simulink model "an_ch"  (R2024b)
settings: Solver=ode45  StartTime=0.0  StopTime=2  MaxStep=.01  RelTol=1e-3  AbsTol=1e-3  EnableMultiTasking=on
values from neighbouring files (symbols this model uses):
  den = 1    [ass_appr.m]    (also in simplify.m = a(find(a):max(size(a))); ass_sis.m; ass1_sis.m; myfbode.m = b)
  den_c = 1    [ass_c.m]    (also in ass_sis.m; ass2_cn.m; ass1_sis.m)
  num = b(find(b):max(size(b)))    [simplify.m]    (also in ass_sis.m = 0; ass1_sis.m = 0; myfbode.m = a; mynyq.m = a)
  num_c = 0    [ass_c.m]    (also in ass_sis.m; ass2_cn.m; ass1_sis.m)
  T = 0; end    [ass_appr.m]    (also in ass_sis.m = 0; ass1_sis.m = 0; myfbode.m = rit)
undefined symbols (not defined in the file or in its folder): sfunyst

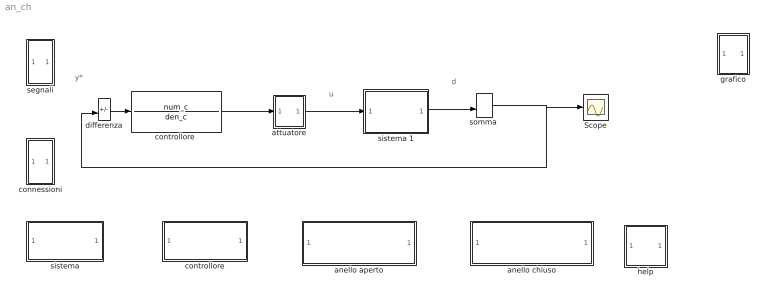
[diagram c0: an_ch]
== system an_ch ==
  note: u
  note: d
  note: y*
  Scope : Scope
  anello aperto : Subsystem
  anello chiuso : Subsystem
  attuatore : Subsystem  mask{upperlimit=inf, lowerlimit=-inf}
      mask prompts: upperlimit "limite superiore"; lowerlimit "limite inferiore"
  connessioni : Subsystem
  controllore : Subsystem
  "controllore " : TransferFcn  Numerator=num_c  Denominator=den_c
  differenza : Sum  Inputs=+-  InputSameDT=on  SaturateOnIntegerOverflow=on
  grafico : Subsystem  Commented=on  mask(Storage scope.){MaskParam1=2, MaskParam2=-10, MaskParam3=10, npts=2000, color='b-/r-/c-./w:/m*/ro/b+'}
      mask prompts: MaskParam1 "Initial Time Range:"; MaskParam2 "Initial y-min:"; MaskParam3 "Initial y-max:"; npts "Storage pts.:"; color "Line type (rgbw-.:xo):"
      mask help: Storage scope using MATLAB graph window. Enter plotting ranges and line type.
      mask init:
      | ax = [0, MaskParam1, MaskParam2, MaskParam3]; dt=-1;
  help : Subsystem
  segnali : Subsystem
  sistema : Subsystem
  sistema 1 : Subsystem
  "somma " : Sum  InputSameDT=on  SaturateOnIntegerOverflow=on
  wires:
  sistema 1/1(out_1) -> "somma "/2
  differenza/1 -> "controllore "/1
  "controllore "/1 -> attuatore/1(In1)
  attuatore/1(Out1) -> sistema 1/1(in_1)
  "somma "/1 -> Scope/1, differenza/2

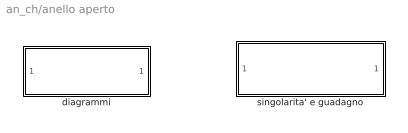
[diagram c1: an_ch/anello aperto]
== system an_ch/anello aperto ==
  diagrammi : Subsystem
  singolarita' e guadagno : Subsystem  mask(singolarita' della f.d.t.){}

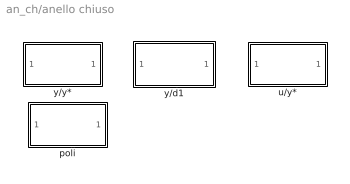
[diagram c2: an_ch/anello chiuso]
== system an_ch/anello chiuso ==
  poli : Subsystem  mask(singolarita' della f.d.t.){}
  u/y* : Subsystem
  y/d1 : Subsystem
  y/y* : Subsystem

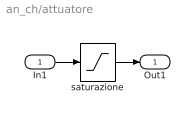
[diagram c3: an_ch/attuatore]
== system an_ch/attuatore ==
  In1 : Inport
  saturazione : Saturate  UpperLimit=upperlimit  LowerLimit=lowerlimit
  Out1 : Outport  VectorParamsAs1DForOutWhenUnconnected=off
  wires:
  saturazione/1 -> Out1/1
  In1/1 -> saturazione/1

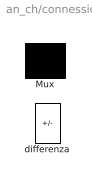
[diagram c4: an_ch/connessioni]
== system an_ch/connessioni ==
  Mux : Mux  Inputs=2
  differenza : Sum  Inputs=+-  InputSameDT=on  SaturateOnIntegerOverflow=on

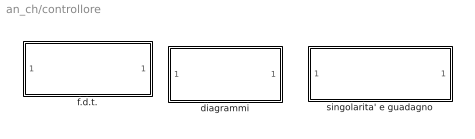
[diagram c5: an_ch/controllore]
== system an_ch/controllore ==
  diagrammi : Subsystem
  f.d.t. : Subsystem  mask(assegnamento controllore){}
  singolarita' e guadagno : Subsystem  mask(singolarita' della f.d.t.){}

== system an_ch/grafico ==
  x : Inport
  "S-function M-file which plots lines " : S-Function  LoadFcn=sfunyst([],[],[],'LoadBlock')  FunctionName=sfunyst  Parameters=ax, color, npts, dt  SFunctionDeploymentMode=off  EnableBusSupport=off
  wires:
  x/1 -> "S-function M-file which plots lines "/1

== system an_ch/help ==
  note: i blocchi con l'ombreggiatura consentono
  note: - l'inserimento della funzione di trasferimento
  note: - l'ottenimento dei diagrammi di Bode e di Nyquist
  note: - la determinazione delle singolarità (poli e/o zeri) e/o del guadagno

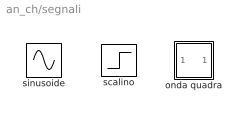
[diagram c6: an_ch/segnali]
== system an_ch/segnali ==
  onda quadra : Subsystem  mask(Pulse Generator){Ts=2, du=1, ht=1, stt=0}
      mask prompts: Ts "Pulse period (secs):"; du "Pulse width:"; ht "Pulse height:"; stt "Pulse start time:"
      mask help: Pulse Generator.
      mask init:
      | ini=ones(length(ht),1); st1=rem(stt,Ts); st2=rem(stt+du,Ts);if(Ts<=1.2*du),ini=zeros(length(ht),1);end;
  scalino : Step  Time=0
  sinusoide : Sin

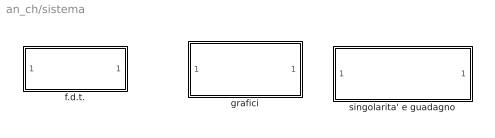
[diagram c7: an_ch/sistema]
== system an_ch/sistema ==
  f.d.t. : Subsystem  mask(assegnamento sistema){}
  grafici : Subsystem
  singolarita' e guadagno : Subsystem  mask(singolarita' della f.d.t.){}

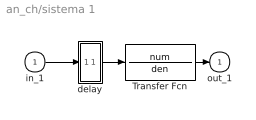
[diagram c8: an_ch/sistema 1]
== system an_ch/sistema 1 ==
  in_1 : Inport
  Transfer Fcn : TransferFcn  Numerator=num  Denominator=den
  delay : Subsystem
  out_1 : Outport  VectorParamsAs1DForOutWhenUnconnected=off
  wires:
  Transfer Fcn/1 -> out_1/1
  in_1/1 -> delay/1(in_1)
  delay/1(out_1) -> Transfer Fcn/1

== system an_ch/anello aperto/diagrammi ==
  Bode : Subsystem
  Nyquist : Subsystem

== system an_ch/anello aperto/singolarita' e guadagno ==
  note: assegna

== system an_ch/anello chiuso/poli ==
  note: assegna

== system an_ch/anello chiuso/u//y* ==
  note: bode

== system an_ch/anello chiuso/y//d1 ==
  note: bode

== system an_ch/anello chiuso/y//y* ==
  note: bode

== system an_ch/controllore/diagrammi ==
  Subsystem1 : Subsystem
  Subsystem2 : Subsystem

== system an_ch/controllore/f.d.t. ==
  note: assegna

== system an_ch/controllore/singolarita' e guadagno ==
  note: assegna

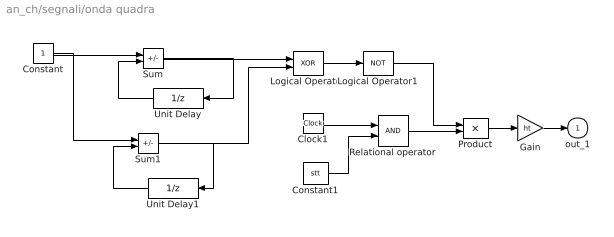
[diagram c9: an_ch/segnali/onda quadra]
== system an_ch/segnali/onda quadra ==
  Clock1 : Clock
  Constant : Constant
  Constant1 : Constant  Value=stt
  Gain : Gain  Gain=ht  SaturateOnIntegerOverflow=on
  Logical Operator : Logic  Operator=XOR
  Logical Operator1 : Logic  Operator=NOT  Inputs=1
  Product : Product  InputSameDT=on  RndMeth=Zero  SaturateOnIntegerOverflow=on
  Relational operator : RelationalOperator
  Sum : Sum  Inputs=+-  InputSameDT=on  SaturateOnIntegerOverflow=on
  Sum1 : Sum  Inputs=+-  InputSameDT=on  SaturateOnIntegerOverflow=on
  Unit Delay : UnitDelay  SampleTime=[Ts,st1]  HasFrameUpgradeWarning=on
  Unit Delay1 : UnitDelay  InitialCondition=ini  SampleTime=[Ts,st2]  HasFrameUpgradeWarning=on
  out_1 : Outport  VectorParamsAs1DForOutWhenUnconnected=off
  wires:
  Logical Operator1/1 -> Product/1
  Logical Operator/1 -> Logical Operator1/1
  Constant1/1 -> Relational operator/2
  Gain/1 -> out_1/1
  Product/1 -> Gain/1
  Relational operator/1 -> Product/2
  Clock1/1 -> Relational operator/1
  Unit Delay/1 -> Sum/2
  Unit Delay1/1 -> Sum1/2
  Constant/1 -> Sum/1, Sum1/1
  Sum/1 -> Unit Delay/1, Logical Operator/1
  Sum1/1 -> Unit Delay1/1, Logical Operator/2

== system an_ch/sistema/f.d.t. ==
  note: assegna

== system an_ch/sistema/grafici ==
  Subsystem1 : Subsystem
  Subsystem2 : Subsystem

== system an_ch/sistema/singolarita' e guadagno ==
  note: assegna

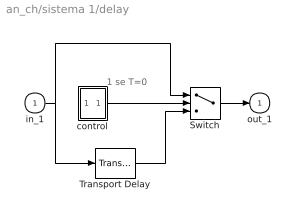
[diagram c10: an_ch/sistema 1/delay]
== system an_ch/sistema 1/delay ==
  note: 1 se T=0
  in_1 : Inport
  Switch : Switch  Threshold=.5
  Transport Delay : TransportDelay  DelayTime=T
  control : Subsystem
  out_1 : Outport  VectorParamsAs1DForOutWhenUnconnected=off
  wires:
  Transport Delay/1 -> Switch/3
  in_1/1 -> Switch/1, Transport Delay/1
  Switch/1 -> out_1/1
  control/1(out_1) -> Switch/2

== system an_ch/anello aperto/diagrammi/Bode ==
  note: bode

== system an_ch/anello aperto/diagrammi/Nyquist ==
  note: bode

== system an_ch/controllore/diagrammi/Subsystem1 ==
  note: bode

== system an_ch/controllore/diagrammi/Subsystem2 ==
  note: bode

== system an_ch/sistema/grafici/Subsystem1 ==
  note: bode

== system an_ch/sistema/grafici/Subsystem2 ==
  note: bode

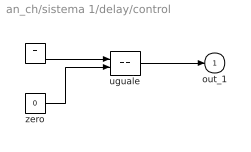
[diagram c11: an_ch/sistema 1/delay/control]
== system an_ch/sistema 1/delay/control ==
  T : Constant  Value=T
  uguale : RelationalOperator  Operator===
  zero : Constant  Value=0
  out_1 : Outport  VectorParamsAs1DForOutWhenUnconnected=off
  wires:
  zero/1 -> uguale/2
  T/1 -> uguale/1
  uguale/1 -> out_1/1
